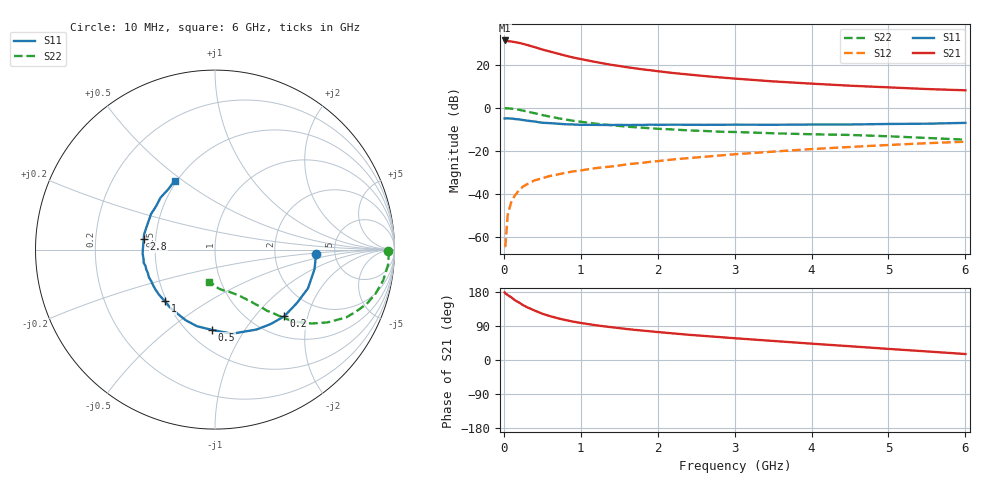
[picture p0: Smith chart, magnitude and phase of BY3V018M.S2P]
! SIEMENS Small Signal Semiconductors
! BFY420
! Si NPN RF SIEGET Grounded Emitter Transistor in MICRO-X
! VCE = 3 V  IC = 18 mA
! Common Emitter S-Parameters:  October  1996
# GHz  S  MA  R  50
!  f  S11  S21  S12  S22
! GHz  MAG  ANG  MAG  ANG  MAG  ANG  MAG  ANG
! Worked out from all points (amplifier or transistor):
!   36 points, 10 MHz to 6 GHz, reference 50 ohm
!   highest |S21| = 31.3 dB at 10 MHz (marker M1)
!   |S21| within 3 dB of that: start of sweep to 389.8 MHz
!   unconditionally stable (mu >= 1): start of sweep to 17.68 MHz; 2.052 GHz to end of sweep
!   at 250 MHz: K = 0.28, MSG = 33.2 dB, |S12| = -36.7 dB
!   at 1.4 GHz: K = 0.89, MSG = 23.7 dB, |S12| = -27.3 dB
!   at 6 GHz: K = 1.07, MAG = 10.3 dB, |S12| = -15.8 dB
!   S11 on the Smith chart (normalised r, x): 10 MHz: 3.58, -0.26; 200 MHz: 1.38, -1.44; 500 MHz: 0.65, -0.73; 1 GHz: 0.49, -0.34; 2.8 GHz: 0.43, +0.06; 6 GHz: 0.49, +0.47
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0.01  0.565 -2.5  36.89 178.4  0.0006 88.9  0.965 -0.5
0.02  0.5629 -4.7  36.57 175.7  0.0006 88.9  0.9681 -1.6
0.05  0.5651 -11.2  35.55 171.5  0.0032 84.1  0.9681 -4.9
0.1  0.5612 -22.7  34.87 164.9  0.0068 76.6  0.9528 -10.4
0.15  0.5447 -33.2  33.56 157.0  0.0094 75.4  0.9278 -15.3
0.2  0.5359 -43.9  32.29 151.3  0.0122 73.3  0.8978 -19.7
0.25  0.5178 -53.3  30.72 144.8  0.0147 69.0  0.8575 -23.8
0.3  0.5019 -62.5  29.06 139.4  0.0165 67.0  0.8223 -27.4
0.4  0.4783 -78.5  25.8 130.5  0.0204 62.6  0.7452 -33.0
0.5  0.4477 -92.1  22.7 122.1  0.0229 60.8  0.6779 -37.4
0.6  0.4386 -103.2  20.34 115.8  0.0259 58.6  0.6206 -40.7
0.7  0.4261 -112.6  18.26 110.2  0.028 57.7  0.5736 -43.3
0.8  0.4131 -120.9  16.36 105.5  0.0306 56.7  0.5328 -45.2
1  0.4011 -134.1  13.61 97.9  0.0347 56.8  0.4723 -47.9
1.1  0.4006 -140.8  12.55 94.6  0.0371 57.1  0.4479 -49.6
1.6  0.3961 -160.9  8.796 81.7  0.0482 56.8  0.3637 -54.5
2.2  0.4039 -176.6  6.449 70.2  0.0626 55.9  0.3123 -59.5
2.8  0.4017 171.6  5.111 60.5  0.0773 53.2  0.2774 -64.2
3.5  0.4018 159.3  4.113 50.3  0.0953 49.4  0.2549 -69.5
4.5  0.4078 143.6  3.265 36.3  0.1223 41.9  0.233 -78.1
5.5  0.4257 127.6  2.728 22.6  0.1497 33.3  0.1983 -91.1
6  0.4452 120.2  2.549 15.8  0.1623 28.6  0.1808 -99.8
